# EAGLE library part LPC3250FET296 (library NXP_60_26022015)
16/32-bit ARM microcontrollers; hardware floating-point coprocessor, USB On-The-Go, and EMC memory interface The LPC3220/30/40/50 embedded microcontrollers were designed for low power, high performance applications. NXP achieved their performance goals using a 90 nanometer process to implement an ARM926EJ-S CPU core with a vector floating point co-processor and a large set of standard peripherals including USB On-The-Go. The LPC3220/30/40/50 operates at CPU frequencies of up to 266 MHz. The NXP implementation uses a ARM926EJ-S CPU core with a Harvard architecture, 5-stage pipeline, and an integral Memory Management Unit (MMU). The MMU provides the virtual memory capabilities needed to support the multi-programming demands of modern operating systems. The ARM926EJ-S also has a hardware based set of DSP instruction extensions, which includes single cycle MAC operations, and hardware based native Jazelle Java Byte-code execution. The NXP implementation has a 32 kB instruction cache and a 32 kB data cache. For low power consumption, the LPC3220/30/40/50 takes advantage of NXP’s advanced technology development to optimize intrinsic power and uses software controlled architectural enhancements to optimize application based power management. The LPC3220/30/40/50 also includes 256 kB of on-chip static RAM, a NAND flash interface, an Ethernet MAC, an LCD controller that supports STN and TFT panels, and an external bus interface that supports SDR and DDR SDRAM as well as static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
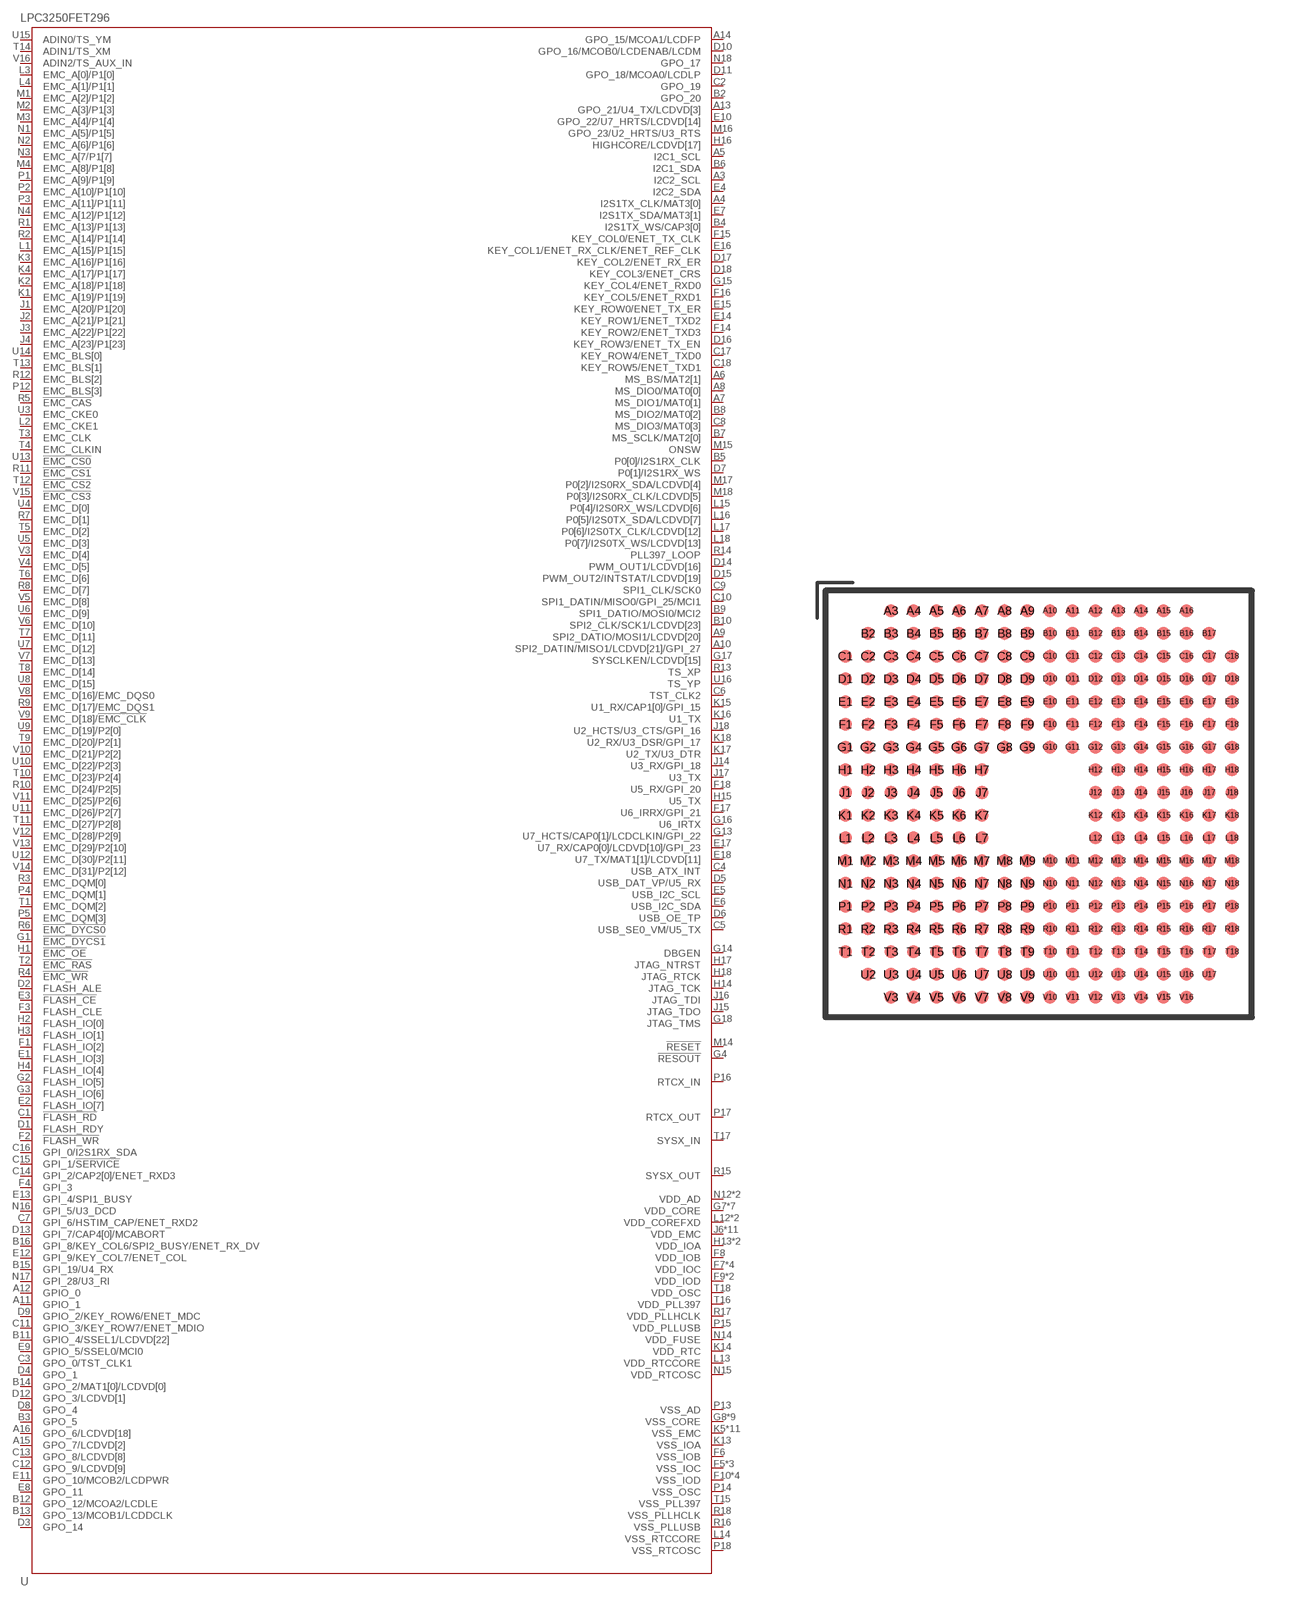
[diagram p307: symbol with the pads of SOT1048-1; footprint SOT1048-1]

Designator prefix U

## LPC3250FET296 (ETHERNET: yes; LCD: yes; SRAM: 256kB)  [SOT1048-1]
A3  I2C2_SCL
A4  I2S1TX_CLK/MAT3[0]
A5  I2C1_SCL
A6  MS_BS/MAT2[1]
A7  MS_DIO1/MAT0[1]
A8  MS_DIO0/MAT0[0]
A9  SPI2_DATIO/MOSI1/LCDVD[20]
A10  SPI2_DATIN/MISO1/LCDVD[21]/GPI_27
A11  GPIO_1
A12  GPIO_0
A13  GPO_21/U4_TX/LCDVD[3]
A14  GPO_15/MCOA1/LCDFP
A15  GPO_7/LCDVD[2]
A16  GPO_6/LCDVD[18]
B2  GPO_20
B3  GPO_5
B4  I2S1TX_WS/CAP3[0]
B5  P0[0]/I2S1RX_CLK
B6  I2C1_SDA
B7  MS_SCLK/MAT2[0]
B8  MS_DIO2/MAT0[2]
B9  SPI1_DATIO/MOSI0/MCI2
B10  SPI2_CLK/SCK1/LCDVD[23]
B11  GPIO_4/SSEL1/LCDVD[22]
B12  GPO_12/MCOA2/LCDLE
B13  GPO_13/MCOB1/LCDDCLK
B14  GPO_2/MAT1[0]/LCDVD[0]
B15  GPI_19/U4_RX
B16  GPI_8/KEY_COL6/SPI2_BUSY/ENET_RX_DV
C1  !FLASH_RD
C2  GPO_19
C3  GPO_0/TST_CLK1
C4  USB_ATX_INT
C5  USB_SE0_VM/U5_TX
C6  TST_CLK2
C7  GPI_6/HSTIM_CAP/ENET_RXD2
C8  MS_DIO3/MAT0[3]
C9  SPI1_CLK/SCK0
C10  SPI1_DATIN/MISO0/GPI_25/MCI1
C11  GPIO_3/KEY_ROW7/ENET_MDIO
C12  GPO_9/LCDVD[9]
C13  GPO_8/LCDVD[8]
C14  GPI_2/CAP2[0]/ENET_RXD3
C15  GPI_1/!SERVICE
C16  GPI_0/I2S1RX_SDA
C17  KEY_ROW4/ENET_TXD0
C18  KEY_ROW5/ENET_TXD1
D1  FLASH_RDY
D2  FLASH_ALE
D3  GPO_14
D4  GPO_1
D5  USB_DAT_VP/U5_RX
D6  USB_OE_TP
D7  P0[1]/I2S1RX_WS
D8  GPO_4
D9  GPIO_2/KEY_ROW6/ENET_MDC
D10  GPO_16/MCOB0/LCDENAB/LCDM
D11  GPO_18/MCOA0/LCDLP
D12  GPO_3/LCDVD[1]
D13  GPI_7/CAP4[0]/MCABORT
D14  PWM_OUT1/LCDVD[16]
D15  PWM_OUT2/INTSTAT/LCDVD[19]
D16  KEY_ROW3/ENET_TX_EN
D17  KEY_COL2/ENET_RX_ER
D18  KEY_COL3/ENET_CRS
E1  FLASH_IO[3]
E2  FLASH_IO[7]
E3  !FLASH_CE
E4  I2C2_SDA
E5  USB_I2C_SCL
E6  USB_I2C_SDA
E7  I2S1TX_SDA/MAT3[1]
E8  GPO_11
E9  GPIO_5/SSEL0/MCI0
E10  GPO_22/U7_HRTS/LCDVD[14]
E11  GPO_10/MCOB2/LCDPWR
E12  GPI_9/KEY_COL7/ENET_COL
E13  GPI_4/SPI1_BUSY
E14  KEY_ROW1/ENET_TXD2
E15  KEY_ROW0/ENET_TX_ER
E16  KEY_COL1/ENET_RX_CLK/ENET_REF_CLK
E17  U7_RX/CAP0[0]/LCDVD[10]/GPI_23
E18  U7_TX/MAT1[1]/LCDVD[11]
F1  FLASH_IO[2]
F2  !FLASH_WR
F3  FLASH_CLE
F4  GPI_3
F5  VSS_IOC
F6  VSS_IOB
F7  VDD_IOC
F8  VDD_IOB
F9  VDD_IOD
F10  VSS_IOD
F11  VSS_IOD
F12  VSS_IOD
F13  VDD_IOD
F14  KEY_ROW2/ENET_TXD3
F15  KEY_COL0/ENET_TX_CLK
F16  KEY_COL5/ENET_RXD1
F17  U6_IRRX/GPI_21
F18  U5_RX/GPI_20
G1  !EMC_DYCS1
G2  FLASH_IO[5]
G3  FLASH_IO[6]
G4  !RESOUT
G5  VSS_IOC
G6  VDD_IOC
G7  VDD_CORE
G8  VSS_CORE
G9  VDD_CORE
G10  VSS_CORE
G11  VDD_CORE
G12  VSS_CORE
G13  U7_HCTS/CAP0[1]/LCDCLKIN/GPI_22
G14  DBGEN
G15  KEY_COL4/ENET_RXD0
G16  U6_IRTX
G17  SYSCLKEN/LCDVD[15]
G18  JTAG_TMS
H1  !EMC_OE
H2  FLASH_IO[0]
H3  FLASH_IO[1]
H4  FLASH_IO[4]
H5  VSS_IOC
H6  VDD_IOC
H7  VSS_CORE
H12  VSS_IOD
H13  VDD_IOA
H14  JTAG_TCK
H15  U5_TX
H16  HIGHCORE/LCDVD[17]
H17  JTAG_NTRST
H18  JTAG_RTCK
J1  EMC_A[20]/P1[20]
J2  EMC_A[21]/P1[21]
J3  EMC_A[22]/P1[22]
J4  EMC_A[23]/P1[23]
J5  VDD_IOC
J6  VDD_EMC
J7  VDD_CORE
J12  VDD_CORE
J13  VDD_IOA
J14  U3_RX/GPI_18
J15  JTAG_TDO
J16  JTAG_TDI
J17  U3_TX
J18  U2_HCTS/U3_CTS/GPI_16
K1  EMC_A[19]/P1[19]
K2  EMC_A[18]/P1[18]
K3  EMC_A[16]/P1[16]
K4  EMC_A[17]/P1[17]
K5  VSS_EMC
K6  VDD_EMC
K7  VDD_EMC
K12  VSS_CORE
K13  VSS_IOA
K14  VDD_RTC
K15  U1_RX/CAP1[0]/GPI_15
K16  U1_TX
K17  U2_TX/U3_DTR
K18  U2_RX/U3_DSR/GPI_17
L1  EMC_A[15]/P1[15]
L2  EMC_CKE1
L3  EMC_A[0]/P1[0]
L4  EMC_A[1]/P1[1]
L5  VSS_EMC
L6  VDD_EMC
L7  VSS_CORE
L12  VDD_COREFXD
L13  VDD_RTCCORE
L14  VSS_RTCCORE
L15  P0[4]/I2S0RX_WS/LCDVD[6]
L16  P0[5]/I2S0TX_SDA/LCDVD[7]
L17  P0[6]/I2S0TX_CLK/LCDVD[12]
L18  P0[7]/I2S0TX_WS/LCDVD[13]
M1  EMC_A[2]/P1[2]
M2  EMC_A[3]/P1[3]
M3  EMC_A[4]/P1[4]
M4  EMC_A[8]/P1[8]
M5  VSS_EMC
M6  VDD_EMC
M7  VDD_CORE
M8  VDD_EMC
M9  VSS_CORE
M10  VSS_CORE
M11  VDD_CORE
M12  VSS_CORE
M13  VDD_COREFXD
M14  !RESET
M15  ONSW
M16  GPO_23/U2_HRTS/U3_RTS
M17  P0[2]/I2S0RX_SDA/LCDVD[4]
M18  P0[3]/I2S0RX_CLK/LCDVD[5]
N1  EMC_A[5]/P1[5]
N2  EMC_A[6]/P1[6]
N3  EMC_A[7/P1[7]
N4  EMC_A[12]/P1[12]
N5  VSS_EMC
N6  VSS_EMC
N7  VDD_EMC
N8  VDD_EMC
N9  VDD_EMC
N10  VDD_EMC
N11  VDD_EMC
N12  VDD_AD
N13  VDD_AD
N14  VDD_FUSE
N15  VDD_RTCOSC
N16  GPI_5/U3_DCD
N17  GPI_28/U3_RI
N18  GPO_17
P1  EMC_A[9]/P1[9]
P2  EMC_A[10]/P1[10]
P3  EMC_A[11]/P1[11]
P4  EMC_DQM[1]
P5  EMC_DQM[3]
P6  VSS_EMC
P7  VSS_EMC
P8  VSS_EMC
P9  VSS_EMC
P10  VSS_EMC
P11  VSS_EMC
P12  EMC_BLS[3]
P13  VSS_AD
P14  VSS_OSC
P15  VDD_PLLUSB
P16  RTCX_IN
P17  RTCX_OUT
P18  VSS_RTCOSC
R1  EMC_A[13]/P1[13]
R2  EMC_A[14]/P1[14]
R3  EMC_DQM[0]
R4  !EMC_WR
R5  !EMC_CAS
R6  !EMC_DYCS0
R7  EMC_D[1]
R8  EMC_D[7]
R9  EMC_D[17]/EMC_DQS1
R10  EMC_D[24]/P2[5]
R11  !EMC_CS1
R12  EMC_BLS[2]
R13  TS_XP
R14  PLL397_LOOP
R15  SYSX_OUT
R16  VSS_PLLUSB
R17  VDD_PLLHCLK
R18  VSS_PLLHCLK
T1  EMC_DQM[2]
T2  !EMC_RAS
T3  EMC_CLK
T4  EMC_CLKIN
T5  EMC_D[2]
T6  EMC_D[6]
T7  EMC_D[11]
T8  EMC_D[14]
T9  EMC_D[20]/P2[1]
T10  EMC_D[23]/P2[4]
T11  EMC_D[27]/P2[8]
T12  !EMC_CS2
T13  EMC_BLS[1]
T14  ADIN1/TS_XM
T15  VSS_PLL397
T16  VDD_PLL397
T17  SYSX_IN
T18  VDD_OSC
U3  EMC_CKE0
U4  EMC_D[0]
U5  EMC_D[3]
U6  EMC_D[9]
U7  EMC_D[12]
U8  EMC_D[15]
U9  EMC_D[19]/P2[0]
U10  EMC_D[22]/P2[3]
U11  EMC_D[26]/P2[7]
U12  EMC_D[30]/P2[11]
U13  !EMC_CS0
U14  EMC_BLS[0]
U15  ADIN0/TS_YM
U16  TS_YP
V3  EMC_D[4]
V4  EMC_D[5]
V5  EMC_D[8]
V6  EMC_D[10]
V7  EMC_D[13]
V8  EMC_D[16]/EMC_DQS0
V9  EMC_D[18]/!EMC_CLK
V10  EMC_D[21]/P2[2]
V11  EMC_D[25]/P2[6]
V12  EMC_D[28]/P2[9]
V13  EMC_D[29]/P2[10]
V14  EMC_D[31]/P2[12]
V15  !EMC_CS3
V16  ADIN2/TS_AUX_IN

## Footprint SOT1048-1 (pad centres in mm)
SOT1048-1 TFBGA296: plastic thin fine-pitch ball grid array package; 296 balls JEDEC: -- IEC: -- JEITA: MO-216
smd 0.45 x 0.45: A3 -5.2,6.8; A4 -4.4,6.8; A5 -3.6,6.8; A6 -2.8,6.8; A7 -2,6.8; A8 -1.2,6.8; A9 -0.4,6.8; A10 0.4,6.8; A11 1.2,6.8; A12 2,6.8; A13 2.8,6.8; A14 3.6,6.8; A15 4.4,6.8; A16 5.2,6.8; B2 -6,6; B3 -5.2,6; B4 -4.4,6; B5 -3.6,6; B6 -2.8,6; B7 -2,6; B8 -1.2,6; B9 -0.4,6; B10 0.4,6; B11 1.2,6; B12 2,6; B13 2.8,6; B14 3.6,6; B15 4.4,6; B16 5.2,6; B17 6,6; C1 -6.8,5.2; C2 -6,5.2; C3 -5.2,5.2; C4 -4.4,5.2; C5 -3.6,5.2; C6 -2.8,5.2; C7 -2,5.2; C8 -1.2,5.2; C9 -0.4,5.2; C10 0.4,5.2; C11 1.2,5.2; C12 2,5.2; C13 2.8,5.2; C14 3.6,5.2; C15 4.4,5.2; C16 5.2,5.2; C17 6,5.2; C18 6.8,5.2; D1 -6.8,4.4; D2 -6,4.4; D3 -5.2,4.4; D4 -4.4,4.4; D5 -3.6,4.4; D6 -2.8,4.4; D7 -2,4.4; D8 -1.2,4.4; D9 -0.4,4.4; D10 0.4,4.4; D11 1.2,4.4; D12 2,4.4; D13 2.8,4.4; D14 3.6,4.4; D15 4.4,4.4; D16 5.2,4.4; D17 6,4.4; D18 6.8,4.4; E1 -6.8,3.6; E2 -6,3.6; E3 -5.2,3.6; E4 -4.4,3.6; E5 -3.6,3.6; E6 -2.8,3.6; E7 -2,3.6; E8 -1.2,3.6; E9 -0.4,3.6; E10 0.4,3.6; E11 1.2,3.6; E12 2,3.6; E13 2.8,3.6; E14 3.6,3.6; E15 4.4,3.6; E16 5.2,3.6; E17 6,3.6; E18 6.8,3.6; F1 -6.8,2.8; F2 -6,2.8; F3 -5.2,2.8; F4 -4.4,2.8; F5 -3.6,2.8; F6 -2.8,2.8; F7 -2,2.8; F8 -1.2,2.8; F9 -0.4,2.8; F10 0.4,2.8; F11 1.2,2.8; F12 2,2.8; F13 2.8,2.8; F14 3.6,2.8; F15 4.4,2.8; F16 5.2,2.8; F17 6,2.8; F18 6.8,2.8; G1 -6.8,2; G2 -6,2; G3 -5.2,2; G4 -4.4,2; G5 -3.6,2; G6 -2.8,2; G7 -2,2; G8 -1.2,2; G9 -0.4,2; G10 0.4,2; G11 1.2,2; G12 2,2; G13 2.8,2; G14 3.6,2; G15 4.4,2; G16 5.2,2; G17 6,2; G18 6.8,2; H1 -6.8,1.2; H2 -6,1.2; H3 -5.2,1.2; H4 -4.4,1.2; H5 -3.6,1.2; H6 -2.8,1.2; H7 -2,1.2; H12 2,1.2; H13 2.8,1.2; H14 3.6,1.2; H15 4.4,1.2; H16 5.2,1.2; H17 6,1.2; H18 6.8,1.2; J1 -6.8,0.4; J2 -6,0.4; J3 -5.2,0.4; J4 -4.4,0.4; J5 -3.6,0.4; J6 -2.8,0.4; J7 -2,0.4; J12 2,0.4; J13 2.8,0.4; J14 3.6,0.4; J15 4.4,0.4; J16 5.2,0.4; J17 6,0.4; J18 6.8,0.4; K1 -6.8,-0.4; K2 -6,-0.4; K3 -5.2,-0.4; K4 -4.4,-0.4; K5 -3.6,-0.4; K6 -2.8,-0.4; K7 -2,-0.4; K12 2,-0.4; K13 2.8,-0.4; K14 3.6,-0.4; K15 4.4,-0.4; K16 5.2,-0.4; K17 6,-0.4; K18 6.8,-0.4; L1 -6.8,-1.2; L2 -6,-1.2; L3 -5.2,-1.2; L4 -4.4,-1.2; L5 -3.6,-1.2; L6 -2.8,-1.2; L7 -2,-1.2; L12 2,-1.2; L13 2.8,-1.2; L14 3.6,-1.2; L15 4.4,-1.2; L16 5.2,-1.2; L17 6,-1.2; L18 6.8,-1.2; M1 -6.8,-2; M2 -6,-2; M3 -5.2,-2; M4 -4.4,-2; M5 -3.6,-2; M6 -2.8,-2; M7 -2,-2; M8 -1.2,-2; M9 -0.4,-2; M10 0.4,-2; M11 1.2,-2; M12 2,-2; M13 2.8,-2; M14 3.6,-2; M15 4.4,-2; M16 5.2,-2; M17 6,-2; M18 6.8,-2; N1 -6.8,-2.8; N2 -6,-2.8; N3 -5.2,-2.8; N4 -4.4,-2.8; N5 -3.6,-2.8; N6 -2.8,-2.8; N7 -2,-2.8; N8 -1.2,-2.8; N9 -0.4,-2.8; N10 0.4,-2.8; N11 1.2,-2.8; N12 2,-2.8; N13 2.8,-2.8; N14 3.6,-2.8; N15 4.4,-2.8; N16 5.2,-2.8; N17 6,-2.8; N18 6.8,-2.8; P1 -6.8,-3.6; P2 -6,-3.6; P3 -5.2,-3.6; P4 -4.4,-3.6; P5 -3.6,-3.6; P6 -2.8,-3.6; P7 -2,-3.6; P8 -1.2,-3.6; P9 -0.4,-3.6; P10 0.4,-3.6; P11 1.2,-3.6; P12 2,-3.6; P13 2.8,-3.6; P14 3.6,-3.6; P15 4.4,-3.6; P16 5.2,-3.6; P17 6,-3.6; P18 6.8,-3.6; R1 -6.8,-4.4; R2 -6,-4.4; R3 -5.2,-4.4; R4 -4.4,-4.4; R5 -3.6,-4.4; R6 -2.8,-4.4; R7 -2,-4.4; R8 -1.2,-4.4; R9 -0.4,-4.4; R10 0.4,-4.4; R11 1.2,-4.4; R12 2,-4.4; R13 2.8,-4.4; R14 3.6,-4.4; R15 4.4,-4.4; R16 5.2,-4.4; R17 6,-4.4; R18 6.8,-4.4; T1 -6.8,-5.2; T2 -6,-5.2; T3 -5.2,-5.2; T4 -4.4,-5.2; T5 -3.6,-5.2; T6 -2.8,-5.2; T7 -2,-5.2; T8 -1.2,-5.2; T9 -0.4,-5.2; T10 0.4,-5.2; T11 1.2,-5.2; T12 2,-5.2; T13 2.8,-5.2; T14 3.6,-5.2; T15 4.4,-5.2; T16 5.2,-5.2; T17 6,-5.2; T18 6.8,-5.2; U2 -6,-6; U3 -5.2,-6; U4 -4.4,-6; U5 -3.6,-6; U6 -2.8,-6; U7 -2,-6; U8 -1.2,-6; U9 -0.4,-6; U10 0.4,-6; U11 1.2,-6; U12 2,-6; U13 2.8,-6; U14 3.6,-6; U15 4.4,-6; U16 5.2,-6; U17 6,-6; V3 -5.2,-6.8; V4 -4.4,-6.8; V5 -3.6,-6.8; V6 -2.8,-6.8; V7 -2,-6.8; V8 -1.2,-6.8; V9 -0.4,-6.8; V10 0.4,-6.8; V11 1.2,-6.8; V12 2,-6.8; V13 2.8,-6.8; V14 3.6,-6.8; V15 4.4,-6.8; V16 5.2,-6.8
